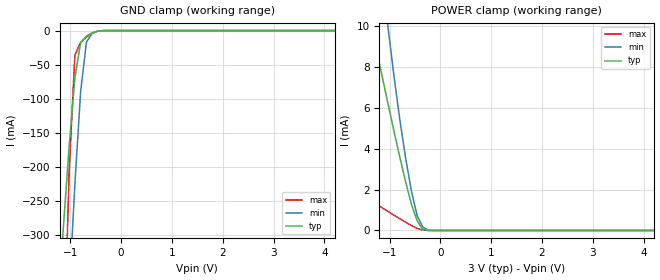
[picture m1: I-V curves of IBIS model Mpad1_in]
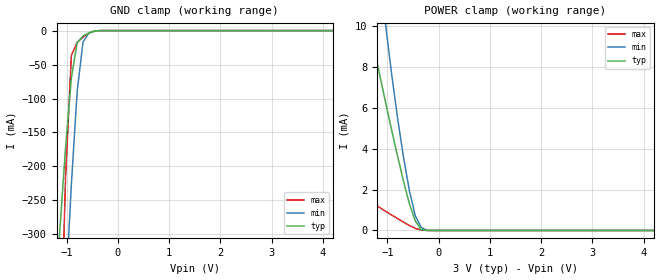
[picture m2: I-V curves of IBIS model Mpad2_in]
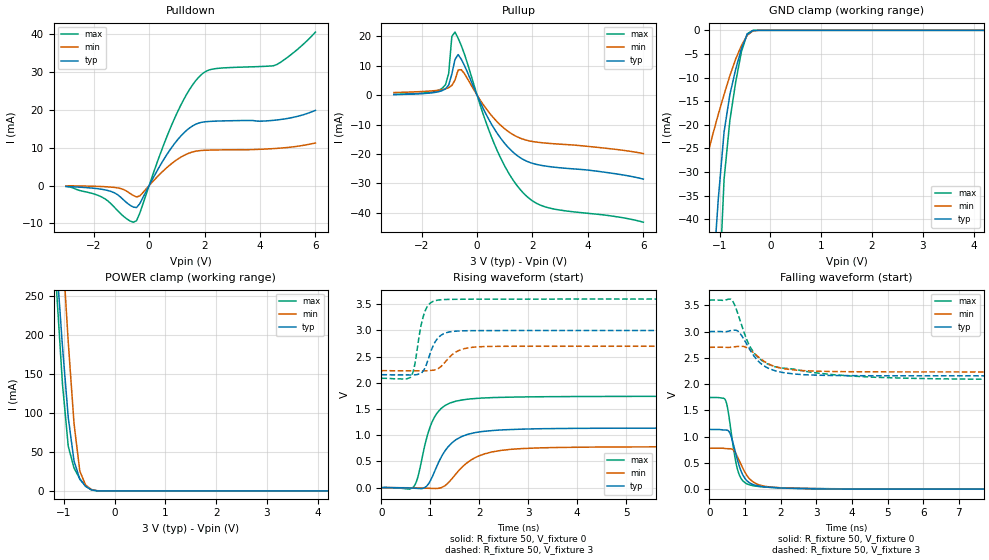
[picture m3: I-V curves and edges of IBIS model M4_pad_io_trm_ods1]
| Created by SiliconSmart  O-2018.09-SP2-3
[IBIS Ver]   4.0
[File Name]   as3316bc.ibs
[File Rev]   1.2
[Date]   Tuesday July 18 2023
|[Source]   Avalanche Team
|[Notes]   Generated IBIS models from Silicon Smart
|[Rev 1.0]  Initial Release based on extracted netlist
|   Characterization
|[Rev 1.1]  Recharacterization with Hspice, run in high accuracy mode
|[Rev 1.2]  Recharacterization with Hspice, align with datasheet parameter
|[Disclaimer]   THE MODEL LIBRARIES ARE PROVIDED AS IS.
|[Copyright]   Copyright 2019, Avalanche Technology., All Rights Reserved
[Component]   as30xx316_BGA
[Manufacturer] Avalanche Technology
| CONTENT :
| This file contains IBIS MODEL for PSRAM device
| AS3032316
| USAGE :
| The models are derived for the 2.7V to 3.6V I/O Operation.
| Temperatures for model generation: typ: 25, max: -40, min: 105
| Voltages : typ: 3.0V, min: 2.7V, max: 3.6V
| PACKAGES SUPPORTED :
| 48-ball FBGA (10mm x 10mm)
| VERIFICATION
| Errors  : 0
| Warnings: 11
| All warnings due to non-monotonic data:
[Package]
R_pkg   0   0 0
L_pkg   0   0 0
C_pkg   0   0 0
[Pin]   signal_name   model_name R_pin   L_pin   C_pin
ADR20   adr_pad_20   Mpad1_in   0.143	2.306E-09	1.043E-12
ADR19   adr_pad_19   Mpad1_in   0.077	1.407E-09	7.164E-13
ADR18   adr_pad_18   Mpad1_in   0.111	1.949E-09	7.824E-13
ADR17   adr_pad_17   Mpad1_in   0.149	2.554E-09	1.099E-12
ADR16   adr_pad_16   Mpad1_in   0.165	2.825E-09	1.197E-12
ADR15   adr_pad_15   Mpad1_in   0.137	2.408E-09	1.144E-12
ADR14   adr_pad_14   Mpad1_in   0.197	3.668E-09	1.21E-12
ADR13   adr_pad_13   Mpad1_in   0.617	9.709E-09	3.005E-12
ADR12   adr_pad_12   Mpad1_in   0.559	1.144E-08	3.033E-12
ADR11   adr_pad_11   Mpad1_in   0.514	1.059E-08	2.826E-12
ADR10   adr_pad_10   Mpad1_in   0.513	8.195E-09	2.638E-12
ADR9   adr_pad_9   Mpad1_in   0.634	8.469E-09	2.789E-12
ADR8   adr_pad_8   Mpad1_in   0.623	8.575E-09	2.776E-12
ADR7   adr_pad_7   Mpad1_in   0.188	3.043E-09	1.338E-12
ADR6   adr_pad_6   Mpad1_in   0.154	2.536E-09	1.187E-12
ADR5   adr_pad_5   Mpad1_in   0.167	2.859E-09	1.111E-12
ADR4   adr_pad_4   Mpad1_in   0.215	3.697E-09	1.292E-12
ADR3   adr_pad_3   Mpad1_in   0.221	3.771E-09	1.419E-12
ADR2   adr_pad_2   Mpad1_in   0.273	5.161E-09	1.7E-12
ADR1   adr_pad_1   Mpad1_in   0.245	4.811E-09	1.599E-12
ADR0   adr_pad_0   Mpad1_in   0.247	4.171E-09	1.541E-12
GN   oe_n_pad   Mpad2_in   0.284	4.462E-09	1.682E-12
EN   ce_n_pad   Mpad2_in   0.202	3.378E-09	1.241E-12
WN   we_n_pad   Mpad2_in   0.332	4.968E-09	1.765E-12
UBN   ub_n_pad   Mpad2_in   0.323	5.035E-09	2.093E-12
LBN   lb_n_pad   Mpad2_in   0.278	4.644E-09	1.918E-12
DQ15   dq_pad_15   Mpad_io   0.084	1.484E-09	7.876E-13
DQ14   dq_pad_14   Mpad_io   0.074	1.31E-09	7.009E-13
DQ13   dq_pad_13   Mpad_io   0.110	1.811E-09	8.59E-13
DQ12   dq_pad_12   Mpad_io   0.107	1.699E-09	8.35E-13
DQ11   dq_pad_11   Mpad_io   0.106	1.702E-09	8.465E-13
DQ10   dq_pad_10   Mpad_io   0.110	1.812E-09	8.515E-13
DQ9   dq_pad_9   Mpad_io   0.086	1.465E-09	7.595E-13
DQ8   dq_pad_8   Mpad_io   0.089	1.561E-09	7.825E-13
DQ7   dq_pad_7   Mpad_io   0.273	4.303E-09	1.612E-12
DQ6   dq_pad_6   Mpad_io   0.201	3.115E-09	1.288E-12
DQ5   dq_pad_5   Mpad_io   0.280	4.16E-09	1.793E-12
DQ4   dq_pad_4   Mpad_io   0.114	1.895E-09	8.643E-13
DQ3   dq_pad_3   Mpad_io   0.117	1.957E-09	9.287E-13
DQ2   dq_pad_2   Mpad_io   0.167	2.604E-09	1.109E-12
DQ1   dq_pad_1   Mpad_io   0.158	2.632E-09	1.093E-12
DQ0   dq_pad_0   Mpad_io   0.223	3.547E-09	1.154E-12
VSS   VSS   GND   NA   NA   NA
VCC   VCC   POWER   NA   NA   NA
|[Package Model]   Package model name.  40-char limit.
| (fill in and uncomment to use this section)
| pad_io
[Model Selector] Mpad_io
| Model Description
M4_pad_io_trm_ods1   60 Ohms drv strength
| Models and submodels in the file (3): Mpad1_in (Input), Mpad2_in (Input), M4_pad_io_trm_ods1 (I/O)
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| pad1_in
[Model] Mpad1_in
Model_type Input
Enable   Active-High
Vinl  =  0.6
Vinh  =  2.4
| Capacitance  typ   min   max
C_comp   2.857182e-12   2.353202e-12   3.152994e-12
| Variables   typ   min   max
[GND Clamp Reference]   0   0   0
[POWER Clamp Reference]   3   2.7   3.6
[Pulldown Reference]   0   0   0
[Pullup Reference]   3   2.7   3.6
[Temperature Range]   25   105   -40
[Voltage Range]   3   2.7   3.6
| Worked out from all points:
|   GND clamp passes 1 mA (typ) near -0.47 V on its own axis
|   POWER clamp passes 1 mA (typ) near -0.53 V on its own axis
[GND Clamp]
| Voltage   I(typ)   I(min)   I(max)
-3V       -2.489A    -3.622A    -6.286A
-1.252V   -415.1mA   -737.7mA   -841.9mA
-1.138V   -289.6mA   -559.5mA   -509.9mA
-1.024V   -170.9mA   -387mA     -208.5mA
-910.3mV  -69.58mA   -225.3mA   -35.91mA
-796.6mV  -17.5mA    -88.85mA   -17.44mA
-682.8mV  -8.077mA   -16.84mA   -9.651mA
-569mV    -3.425mA   -3.886mA   -3.679mA
-455.2mV  -663.4uA   -928.9uA   -526.9uA
-227.6mV  -421.5nA   -3.52uA    -35.99nA
6V        0A         0A         0A
[POWER Clamp]
| Voltage   I(typ)   I(min)   I(max)
-3V       32.41mA    56.72mA    4.109mA
-1.366V   10.2mA     17.4mA     1.461mA
-1.252V   8.822mA    14.8mA     1.281mA
-1.024V   6.137mA    9.837mA    922.9uA
-910.3mV  4.838mA    7.526mA    746.6uA
-796.6mV  3.581mA    5.417mA    573.1uA
-682.8mV  2.387mA    3.545mA    403.9uA
-569mV    1.291mA    1.93mA     242.9uA
-455.2mV  467.9uA    721.2uA    103.5uA
-341.4mV  48.97uA    156.2uA    20.84uA
-113.8mV  7.993nA    354.4nA    880.4pA
6V        0A         0A         0A
| pad2_in
[Model] Mpad2_in
Model_type Input
Enable   Active-High
Vinl  =  0.6
Vinh  =  2.4
| Capacitance  typ   min   max
C_comp   2.865723e-12   2.362138e-12   3.161751e-12
| Variables   typ   min   max
[GND Clamp Reference]   0   0   0
[POWER Clamp Reference]   3   2.7   3.6
[Pulldown Reference]   0   0   0
[Pullup Reference]   3   2.7   3.6
[Temperature Range]   25   105   -40
[Voltage Range]   3   2.7   3.6
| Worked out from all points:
|   GND clamp passes 1 mA (typ) near -0.47 V on its own axis
|   POWER clamp passes 1 mA (typ) near -0.53 V on its own axis
[GND Clamp]
| Voltage   I(typ)   I(min)   I(max)
-3V       -2.583A    -3.873A    -6.564A
-1.138V   -296.1mA   -573.1mA   -531mA
-1.024V   -173.3mA   -391.8mA   -216.6mA
-910.3mV  -69.77mA   -226.3mA   -36.44mA
-796.6mV  -17.49mA   -89.03mA   -17.43mA
-682.8mV  -8.073mA   -16.84mA   -9.646mA
-569mV    -3.423mA   -3.884mA   -3.677mA
-455.2mV  -662.9uA   -928.4uA   -526.4uA
-227.6mV  -421nA     -3.517uA   -35.92nA
6V        0A         0A         0A
[POWER Clamp]
| Voltage   I(typ)   I(min)   I(max)
-3V       32.41mA    56.72mA    4.109mA
-1.366V   10.2mA     17.4mA     1.461mA
-1.252V   8.822mA    14.8mA     1.281mA
-1.024V   6.137mA    9.837mA    922.9uA
-910.3mV  4.838mA    7.526mA    746.6uA
-796.6mV  3.581mA    5.417mA    573.1uA
-682.8mV  2.387mA    3.545mA    403.9uA
-569mV    1.291mA    1.93mA     242.9uA
-455.2mV  467.9uA    721.2uA    103.5uA
-341.4mV  48.97uA    156.2uA    20.84uA
-113.8mV  7.993nA    354.4nA    880.4pA
6V        0A         0A         0A
[Model] M4_pad_io_trm_ods1
Model_type I/O
Enable   Active-High
Vinl  =  0.6
Vinh  =  2.4
Vmeas =  1.5
Cref  =  30e-12
| Capacitance  typ   min   max
C_comp   4.118801e-12   3.947848e-12   4.414159e-12
| Variables   typ   min   max
[GND Clamp Reference]   0   0   0
[POWER Clamp Reference]   3   2.7   3.6
[Pulldown Reference]   0   0   0
[Pullup Reference]   3   2.7   3.6
[Temperature Range]   25   105   -40
[Voltage Range]   3   2.7   3.6
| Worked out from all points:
|   slope of the pulldown table from 0 to 0.45 V, typ, clamps not added: 75.6 ohm
|   slope of the pullup table from 0 to 0.45 V, typ, clamps not added: 51.8 ohm
|   GND clamp passes 1 mA (typ) near -0.46 V on its own axis
|   POWER clamp passes 1 mA (typ) near -0.42 V on its own axis
|   falling waveform, R_fixture 50, V_fixture 0: 20-80 % time 325ps typ, 411ps min, 252ps max; typ from 1.14 V to 0 V
|   falling waveform, R_fixture 50, V_fixture 3: 20-80 % time 602ps typ, 661ps min, 794ps max; typ from 3 V to 2.15 V
|   rising waveform, R_fixture 50, V_fixture 0: 20-80 % time 466ps typ, 621ps min, 335ps max; typ from 0 V to 1.14 V
|   rising waveform, R_fixture 50, V_fixture 3: 20-80 % time 225ps typ, 326ps min, 176ps max; typ from 2.15 V to 3 V
[GND Clamp]
| Voltage   I(typ)   I(min)   I(max)
-3V       -379.8mA   -106mA     -725.8mA
-1.593V   -131.7mA   -42.01mA   -247mA
-1.479V   -111.8mA   -36.94mA   -208.5mA
-1.138V   -53.52mA   -22.25mA   -94.22mA
-1.024V   -35.67mA   -17.76mA   -59.08mA
-910.3mV  -21.49mA   -13.58mA   -31.51mA
-796.6mV  -13.6mA    -9.604mA   -19.09mA
-682.8mV  -8.279mA   -6.099mA   -11mA
-569mV    -3.88mA    -3.236mA   -4.53mA
-455.2mV  -866.7uA   -1.043mA   -727.1uA
-341.4mV  -35.72uA   -109.2uA   -11.2uA
6V        0A         0A         0A
[POWER Clamp]
| Voltage   I(typ)   I(min)   I(max)
-3V       2.191A     2.679A     2.475A
-1.138V   291mA      439mA      255.8mA
-1.024V   186.1mA    312.2mA    137.6mA
-910.3mV  94.47mA    191.5mA    57.5mA
-796.6mV  38.47mA    86.67mA    29.42mA
-682.8mV  15.04mA    25.47mA    15.61mA
-569mV    5.939mA    7.524mA    6.125mA
-455.2mV  1.483mA    1.86mA     1.35mA
-227.6mV  1.148uA    12.93uA    332nA
6V        0A         0A         0A
[Pulldown]
| Voltage   I(typ)   I(min)   I(max)
-3V       -248.9uA   -57.27uA   -211.8uA
-1.934V   -763.9uA   -203.6uA   -2.351mA
-1.479V   -1.326mA   -352.6uA   -4.122mA
-796.6mV  -4.614mA   -1.551mA   -8.859mA
-455.2mV  -5.81mA    -3.008mA   -9.281mA
413.8mV   5.511mA    3.198mA    8.617mA
827.6mV   10.2mA     5.892mA    16.24mA
1.345V    14.53mA    8.266mA    23.98mA
1.759V    16.42mA    9.161mA    28.37mA
2.276V    16.97mA    9.375mA    30.72mA
4.614V    17.32mA    9.818mA    31.97mA
6V        19.86mA    11.25mA    40.51mA
[Pullup]
| Voltage   I(typ)   I(min)   I(max)
-3V       187.4uA    871.4uA    220.3uA
-1.252V   1.555mA    1.876mA    2.377mA
-1.024V   3.43mA     2.541mA    7.364mA
-910.3mV  7.139mA    3.267mA    19.92mA
-796.6mV  12.13mA    5.096mA    21.41mA
-682.8mV  13.76mA    8.544mA    19.32mA
-569mV    12.16mA    8.636mA    16.81mA
620.7mV   -11.43mA   -8.01mA    -16.55mA
1.138V    -17.91mA   -12.44mA   -26.44mA
1.655V    -21.81mA   -14.96mA   -33.11mA
2.586V    -24.25mA   -16.39mA   -38.3mA
6V        -28.52mA   -19.85mA   -43.17mA
[Ramp]
dV/dt_r   0.681951/0.465717n  0.468514/0.620601n  1.04707/0.335033n
dV/dt_f   0.507478/0.602469n  0.281038/0.661038n  0.908676/0.793971n
R_load = 50
[Falling Waveform]
R_fixture = 50
V_fixture = 0
V_fixture_min = 0
V_fixture_max = 0
| Time   V(typ)   V(min)   V(max)
0s        1.137V     780.9mV    1.745V
449.9ps   1.126V     772.6mV    1.697V
508.1ps   1.122V     771mV      1.558V
603.1ps   1.02V      768.8mV    1.127V
721ps     726.5mV    702.8mV    590.2mV
828.5ps   459.1mV    557.6mV    291.5mV
1.004ns   198.3mV    313.9mV    120.4mV
1.349ns   64.63mV    94.58mV    52.82mV
3.774ns   2.102mV    4.005mV    6.578mV
21.88ns   -42.85nV   140nV      61.39nV
[Falling Waveform]
R_fixture = 50
V_fixture = 3
V_fixture_min = 2.7
V_fixture_max = 3.6
| Time   V(typ)   V(min)   V(max)
0s        3V         2.7V       3.6V
634.8ps   3.023V     2.703V     3.597V
847.3ps   2.977V     2.719V     3.241V
1.169ns   2.619V     2.638V     2.678V
1.378ns   2.432V     2.516V     2.503V
1.62ns    2.314V     2.399V     2.386V
2.203ns   2.207V     2.282V     2.298V
3.494ns   2.163V     2.239V     2.178V
7.486ns   2.158V     2.232V     2.093V
21.88ns   2.154V     2.232V     2.086V
[Rising Waveform]
R_fixture = 50
V_fixture = 0
V_fixture_min = 0
V_fixture_max = 0
| Time   V(typ)   V(min)   V(max)
0s        24.24nV    299.5nV    41.88nV
653.2ps   -9.927mV   -1.656mV   10.12mV
759.1ps   -16.54mV   -3.819mV   256.1mV
919.1ps   24.84mV    -9.607mV   933.3mV
1.136ns   419.1mV    -14.93mV   1.424V
1.43ns    847.3mV    159.7mV    1.625V
1.82ns    1.031V     521.5mV    1.695V
2.443ns   1.101V     711mV      1.724V
3.955ns   1.132V     771.8mV    1.74V
21.88ns   1.137V     780.9mV    1.745V
[Rising Waveform]
R_fixture = 50
V_fixture = 3
V_fixture_min = 2.7
V_fixture_max = 3.6
| Time   V(typ)   V(min)   V(max)
0s        2.154V     2.232V     2.086V
596.6ps   2.152V     2.231V     2.111V
670.7ps   2.154V     2.231V     2.302V
806.3ps   2.186V     2.231V     3.083V
893ps     2.296V     2.231V     3.375V
1.061ns   2.72V      2.243V     3.558V
1.23ns    2.917V     2.326V     3.588V
1.576ns   2.991V     2.616V     3.596V
2.22ns    2.998V     2.696V     3.598V
21.88ns   3V         2.7V       3.6V
